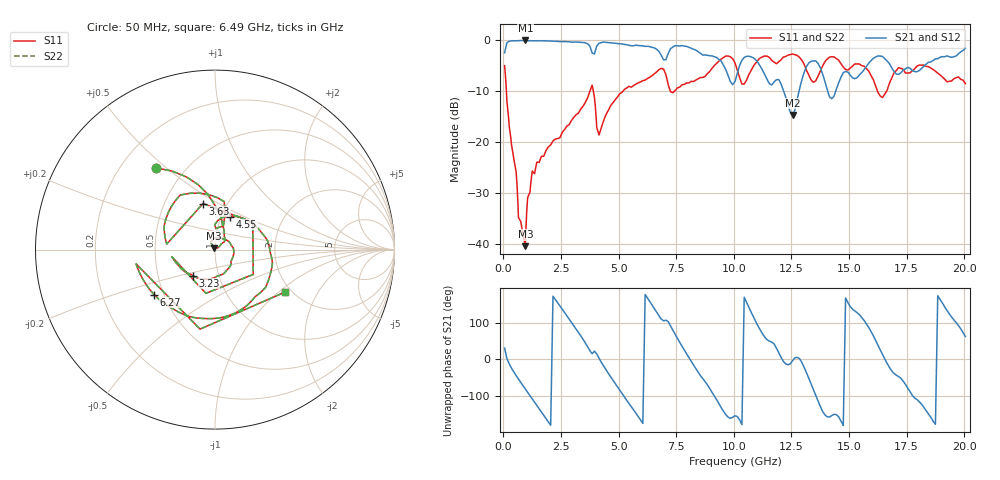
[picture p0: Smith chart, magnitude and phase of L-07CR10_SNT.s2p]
#	mhz	s	ma	r	50
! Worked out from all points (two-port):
!   1001 points, 50 MHz to 20.05 GHz, reference 50 ohm
!   highest |S21| = -0.09 dB at 950 MHz (marker M1); lowest = -14.7 dB at 12.55 GHz (marker M2)
!   |S21| within 3 dB of the highest: start of sweep to 6.861 GHz; 7.113 GHz to 8.955 GHz (1.842 GHz wide, 22.9 % of centre)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
!   lowest |S11| = -40.4 dB at 950 MHz (marker M3), VSWR 1.02, Z = 49.3 + j0.67 ohm
!   |S11| at or under -10 dB: 128.2 MHz to 3.756 GHz (3.628 GHz wide, 187 % of centre); 3.9 GHz to 5.194 GHz (1.293 GHz wide, 28.4 % of centre); 16.23 GHz to 16.64 GHz (404.4 MHz wide, 2.46 % of centre)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
!   |S22| runs from -40.4 to -2.7 dB; largest |S21 - S12| = 0
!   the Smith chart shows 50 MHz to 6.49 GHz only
!   S11 on the Smith chart (normalised r, x): 50 MHz: 0.35, +0.46; 3.23 GHz: 0.75, -0.23; 3.63 GHz: 0.77, +0.43; 4.55 GHz: 1.10, +0.42; 6.27 GHz: 0.44, -0.27; 6.49 GHz: 1.84, -1.10
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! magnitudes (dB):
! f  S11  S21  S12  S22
! 50 MHz  -5.0  -2.5  -2.5  -5.0
! 730 MHz  -35.4  -0.1  -0.1  -35.4
! 950 MHz  -40.4  -0.1  -0.1  -40.4
! 1.35 GHz  -26.2  -0.2  -0.2  -26.2
! 3.23 GHz  -14.4  -0.4  -0.4  -14.4
! 3.39 GHz  -13.4  -0.5  -0.5  -13.4
! 3.63 GHz  -11.5  -0.7  -0.7  -11.5
! 3.87 GHz  -9.3  -2.6  -2.6  -9.3
! 4.15 GHz  -18.6  -0.6  -0.6  -18.6
! 4.55 GHz  -13.9  -0.5  -0.5  -13.9
! 6.27 GHz  -7.5  -1.2  -1.2  -7.5
! 6.49 GHz  -6.8  -1.5  -1.5  -6.8
! 6.73 GHz  -5.9  -2.2  -2.2  -5.9
! 7.35 GHz  -10.3  -1.4  -1.4  -10.3
! 10.05 GHz  -4.5  -8.1  -8.1  -4.5
! 10.81 GHz  -5.4  -3.4  -3.4  -5.4
! 12.55 GHz  -2.7  -14.7  -14.7  -2.7
! 13.39 GHz  -8.0  -4.1  -4.1  -8.0
! 14.25 GHz  -3.3  -11.5  -11.5  -3.3
! 16.73 GHz  -8.8  -4.5  -4.5  -8.8
! 18.15 GHz  -4.9  -5.6  -5.6  -4.9
! 20.05 GHz  -8.5  -1.6  -1.6  -8.5
